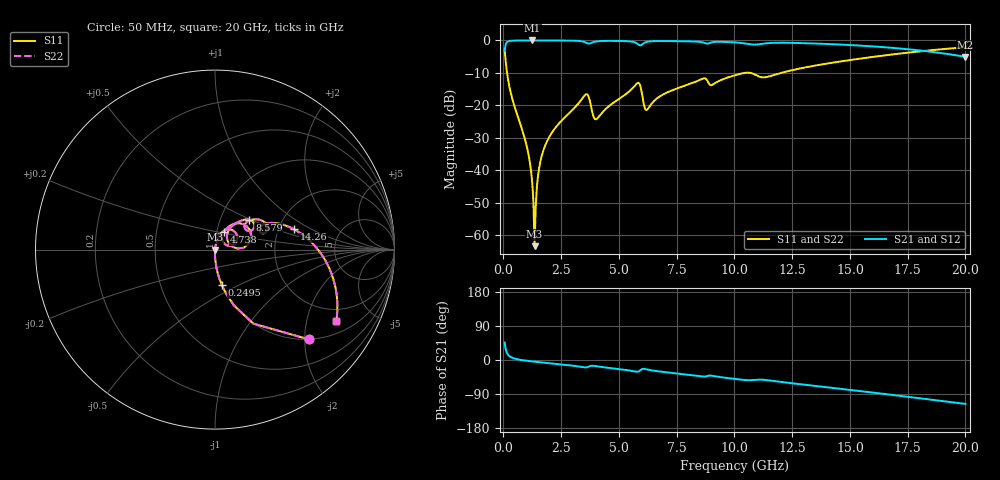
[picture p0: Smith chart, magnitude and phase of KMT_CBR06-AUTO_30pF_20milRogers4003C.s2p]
! Data measured by Modelithics Inc. support@modelithics.com 813-866-6335
! KEMET CBR06-AUTO 30pF, Pad Width= 0.851mm, Pad Length= 0.64mm, Pad Gap= 0.62mm, 20mil Rogers 4003C substrate Data, January 2022
# hz S ma R 50
! 2 Port Network Data from SP1.SP block
! freq  magS11  angS11  magS21  angS21  magS12  angS12  magS22  angS22
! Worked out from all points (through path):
!   401 points, 50 MHz to 20 GHz, reference 50 ohm
!   highest |S21| = -0.01 dB at 1.247 GHz (marker M1); lowest = -5.1 dB at 20 GHz (marker M2)
!   group delay of S21, straight-line fit = 16.2 ps
!   lowest |S11| = -63.3 dB at 1.347 GHz (marker M3), VSWR 1.00, Z = 50.1 - j0.0308 ohm
!   |S11| at or under -10 dB: 156.6 MHz to 10.44 GHz (10.28 GHz wide, 194 % of centre); 10.69 GHz to 12.02 GHz (1.325 GHz wide, 11.7 % of centre)
!   |S22| runs from -63.3 to -2.1 dB; largest |S21 - S12| = 0
!   S11 on the Smith chart (normalised r, x): 50 MHz: 0.99, -2.10; 249.5 MHz: 0.99, -0.41; 4.738 GHz: 1.08, +0.21; 8.579 GHz: 1.37, +0.49; 14.26 GHz: 2.44, +0.69; 20 GHz: 1.46, -3.02
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5e7  0.7248 -43.7  0.6886 46.3  0.6886 46.3  0.7248 -43.7
2.495e8  0.2 -79.2  0.9794 10.7  0.9794 10.7  0.2 -79.2
1.0475e9  0.02036 -90.8  0.9992 -2.4  0.9992 -2.4  0.02036 -90.8
1.197125e9  0.009663 -90.0  0.9993 -3.5  0.9993 -3.5  0.009663 -90.0
1.247e9  0.006423 -88.5  0.9993 -3.8  0.9993 -3.8  0.006423 -88.5
1.34675e9  0.0006803 -26.9  0.9993 -4.5  0.9993 -4.5  0.0006803 -26.9
1.4465e9  0.005522 78.0  0.9993 -5.2  0.9993 -5.2  0.005522 78.0
1.596125e9  0.01356 80.9  0.9991 -6.1  0.9991 -6.1  0.01356 80.9
1.8455e9  0.02603 80.5  0.9988 -7.7  0.9988 -7.7  0.02603 80.5
3.391625e9  0.1247 61.2  0.9698 -18.4  0.9698 -18.4  0.1247 61.2
3.641e9  0.1466 32.3  0.9012 -18.7  0.9012 -18.7  0.1466 32.3
3.990125e9  0.06098 37.2  0.9623 -16.2  0.9623 -16.2  0.06098 37.2
4.73825e9  0.1084 63.0  0.9846 -22.0  0.9846 -22.0  0.1084 63.0
5.785625e9  0.2191 36.9  0.8968 -31.0  0.8968 -31.0  0.2191 36.9
6.184625e9  0.0846 28.6  0.9467 -24.5  0.9467 -24.5  0.0846 28.6
6.73325e9  0.1349 54.8  0.9787 -30.2  0.9787 -30.2  0.1349 54.8
8.578625e9  0.2538 40.9  0.9409 -43.1  0.9409 -43.1  0.2538 40.9
1.0025e10  0.2914 35.3  0.9328 -50.1  0.9328 -50.1  0.2914 35.3
1.336662e10  0.4022 20.2  0.8997 -67.5  0.8997 -67.5  0.4022 20.2
1.426438e10  0.4552 14.3  0.8747 -73.7  0.8747 -73.7  0.4552 14.3
1.670825e10  0.6006 -3.4  0.7757 -91.2  0.7757 -91.2  0.6006 -3.4
2e10  0.7846 -30.5  0.5585 -115.9  0.5585 -115.9  0.7846 -30.5
